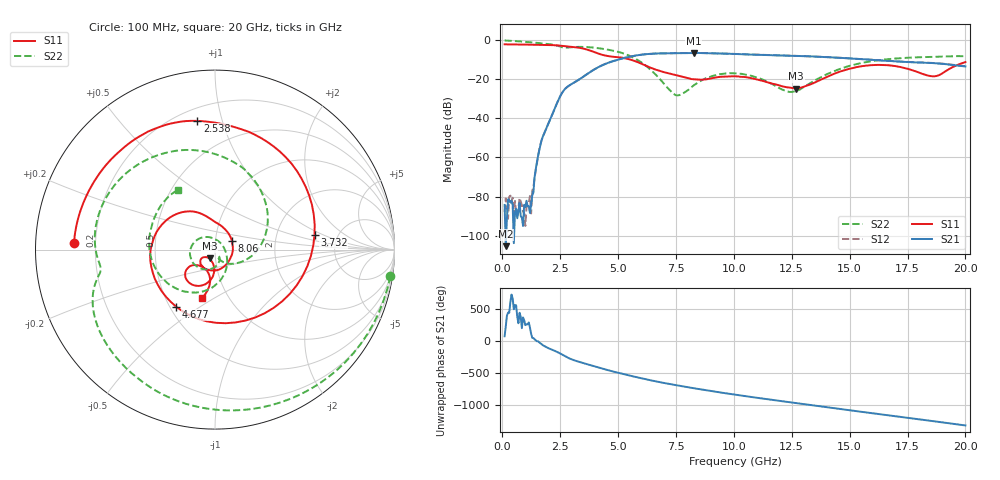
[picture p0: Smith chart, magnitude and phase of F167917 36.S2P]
!  2-Port S-parameters saved by WinCal
! VAR MeasName=S-Parameters (CALIBRATED_DATA) read from VNA (N5242A)
! VAR MeasDate=2016-11-22 9:01:32
! VAR NAME=F167917 36
! VAR FILENAME=F167917 36.S2P
! VAR DATE=2016-11-22 9:01:32
! VAR PHYS_PORTS=1,2
# Hz S DB R 50
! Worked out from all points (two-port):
!   401 points, 100 MHz to 20 GHz, reference 50 ohm
!   highest |S21| = -6.47 dB at 8.259 GHz (marker M1); lowest = -105.4 dB at 149.8 MHz (marker M2)
!   |S21| within 3 dB of the highest: 5.137 GHz to 15.27 GHz (10.13 GHz wide, 99.3 % of centre)
!   lowest |S11| = -24.8 dB at 12.69 GHz (marker M3), VSWR 1.12, Z = 46.8 - j4.57 ohm
!   |S11| at or under -10 dB: 5.561 GHz to end of sweep
!   |S22| runs from -28.2 to -0.1 dB; largest |S21 - S12| = 0.0051
!   S11 on the Smith chart (normalised r, x): 100 MHz: 0.12, +0.02; 2.538 GHz: 0.28, +0.83; 3.732 GHz: 3.35, +0.78; 4.677 GHz: 0.54, -0.40; 8.06 GHz: 1.20, +0.12; 20 GHz: 0.76, -0.44
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1e8  -2.09 177.3  -84.28 75.9  -87.79 23.2  -0.10 -8.7
1.4975e8  -2.09 176.0  -105.39 -132.5  -80.96 17.8  -0.13 -12.8
1.24425e9  -2.26 146.2  -84.13 115.7  -88.64 113.1  -1.06 -94.1
1.692e9  -2.35 132.4  -51.31 -45.4  -51.43 -47.3  -1.57 -121.6
2.53775e9  -2.81 97.9  -27.82 159.2  -27.81 158.9  -3.40 -166.2
3.43325e9  -4.10 39.4  -19.18 24.6  -19.20 24.6  -3.40 161.6
3.73175e9  -5.03 8.2  -16.75 -6.7  -16.76 -6.5  -3.55 147.2
4.22925e9  -7.14 -59.4  -13.28 -58.8  -13.24 -58.6  -4.19 122.3
4.677e9  -8.29 -123.9  -11.12 -103.2  -11.05 -103.4  -5.09 98.5
5.72175e9  -10.63 138.1  -7.89 164.9  -7.90 164.6  -9.26 31.3
6.7665e9  -15.58 95.7  -6.73 83.7  -6.76 83.5  -19.37 -46.7
7.463e9  -17.71 68.0  -6.60 36.8  -6.61 36.8  -27.94 -66.8
8.06e9  -19.48 26.7  -6.48 -0.4  -6.50 -0.3  -25.18 -62.1
8.259e9  -19.96 9.5  -6.47 -12.7  -6.49 -12.5  -23.18 -69.9
1.005e10  -18.40 -118.3  -7.00 -113.6  -7.00 -113.5  -16.95 -165.3
1.129375e10  -20.95 -146.9  -7.53 -176.7  -7.51 -176.7  -20.38 134.3
1.268675e10  -24.82 -122.0  -7.97 115.3  -7.98 115.1  -25.98 15.0
1.338325e10  -22.23 -98.6  -8.28 80.9  -8.27 81.0  -21.36 -37.8
1.497525e10  -14.66 -101.8  -9.30 4.9  -9.26 4.8  -13.18 -96.9
1.67165e10  -12.84 -135.5  -10.57 -76.3  -10.59 -76.4  -9.61 -149.3
1.865675e10  -18.46 -120.8  -11.71 -167.3  -11.67 -167.3  -8.49 159.5
2e10  -11.17 -104.7  -13.41 127.1  -13.27 126.9  -8.15 121.7
